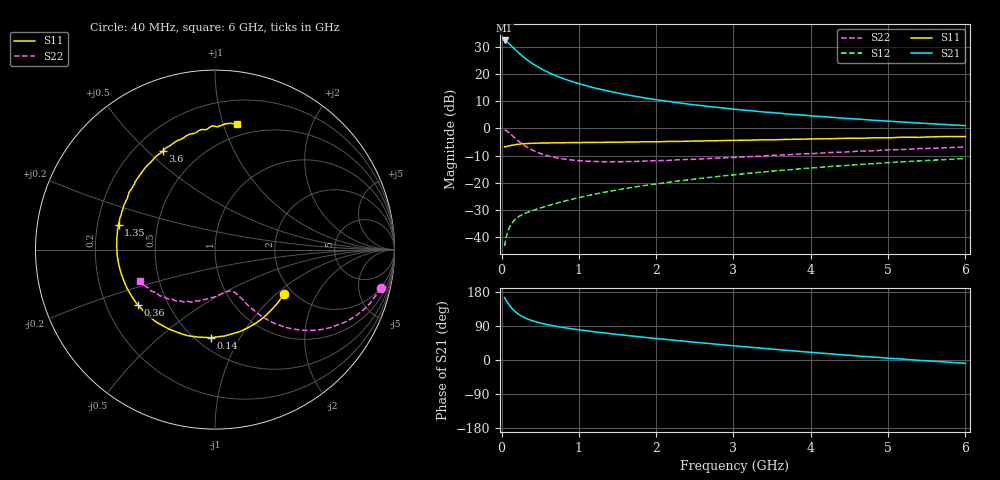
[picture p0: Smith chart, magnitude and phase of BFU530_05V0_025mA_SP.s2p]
! Filename:  P:\Prog\Test\Noise\ATS_data\Testdata_Net\03 Spar\BFU530_APG2013_40_A05_05p0V_025mA_SP_CM01_D.s2p
! Date/Time: Fri 26/Apr/2013 13:03:14
! BFU530_APG2013_40_A05_05p0V_1to25mA_SP_CM01_Bias8_R.s2p
! MDIF S-parameter v. bias file
! BFU530_APG2013_40_A05_05p0V_1to25mA_SP_CM01
! Date/time Wed Apr 24 19:36:53 2013
! VAR V_out= 5.0000
! VAR I_out= 24.9950
! VAR V_in= 0.8387
! VAR I_in= 0.2810
! Device data file deembeded for feedlines and parallel
! Original file: \03 Spar\BFU530_APG2013_40_A05_05p0V_025mA_SP_CM01_R.s2p
! Feed-files: PR047V01_250413_Feed1.s2p, PR047V01_250413_Feed2.s2p
! Parallel-file: PR047V01_250413_Par.s2p
# MHz S MA R 50
!  Freq-MHz  S11-mag  S11-arg  S21-mag  S21-arg  S12-mag  S12-arg  S22-mag  S22-arg
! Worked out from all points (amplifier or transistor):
!   98 points, 40 MHz to 6 GHz, reference 50 ohm
!   highest |S21| = 32.5 dB at 40 MHz (marker M1)
!   |S21| within 3 dB of that: start of sweep to 163.5 MHz
!   unconditionally stable (mu >= 1): 1.114 GHz to 3.212 GHz
!   at 300 MHz: K = 0.54, MSG = 28.7 dB, |S12| = -31.4 dB
!   at 1.6 GHz: K = 1.05, MAG = 16.0 dB, |S12| = -22.2 dB
!   at 6 GHz: K = 0.84, MSG = 6.1 dB, |S12| = -11.1 dB
!   S11 on the Smith chart (normalised r, x): 40 MHz: 1.81, -1.12; 140 MHz: 0.59, -0.76; 360 MHz: 0.34, -0.29; 1.35 GHz: 0.29, +0.12; 3.6 GHz: 0.31, +0.56; 6 GHz: 0.40, +1.11
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40  0.4571 -32.5  42.01 164.5  0.006714 79.4  0.9469 -12.9
50  0.4589 -40.5  41.53 160.4  0.008226 77.0  0.9316 -16.0
80  0.4692 -61.0  38.43 151.0  0.0124 70.0  0.8717 -24.6
90  0.4725 -67.1  37.35 147.9  0.01358 68.0  0.849 -27.1
120  0.4844 -83.5  34.23 139.8  0.0167 63.1  0.7789 -33.8
140  0.491 -92.6  32.13 135.1  0.0184 60.5  0.7339 -37.5
180  0.5034 -107.6  28.24 127.3  0.02128 56.7  0.652 -43.4
200  0.5059 -113.7  26.5 123.9  0.02241 55.3  0.6159 -45.8
240  0.5142 -123.9  23.51 118.2  0.02438 53.6  0.5536 -49.5
300  0.5226 -135.6  19.94 111.6  0.02689 52.4  0.4814 -53.5
360  0.5294 -144.3  17.2 106.5  0.02911 52.2  0.428 -56.3
460  0.5342 -154.8  13.9 99.9  0.03263 53.1  0.3655 -59.1
600  0.5393 -165.3  10.93 93.1  0.03754 55.0  0.3123 -61.4
800  0.5446 -175.5  8.317 85.8  0.04495 57.5  0.2735 -64.2
1050  0.5495 174.7  6.398 78.4  0.05476 59.6  0.2519 -67.8
1350  0.5549 165.7  5.006 71.0  0.0671 60.8  0.2433 -72.6
2050  0.569 148.8  3.305 55.8  0.09646 59.9  0.2545 -86.0
3100  0.6038 126.8  2.203 35.9  0.1436 55.1  0.2971 -106.7
3600  0.6212 117.8  1.906 27.1  0.1674 51.5  0.323 -115.5
4100  0.6429 108.8  1.667 18.8  0.1904 47.7  0.3476 -125.1
5200  0.6897 91.4  1.308 2.4  0.2423 38.2  0.4076 -144.1
6000  0.7084 80.1  1.126 -8.8  0.2778 30.4  0.4553 -157.2
